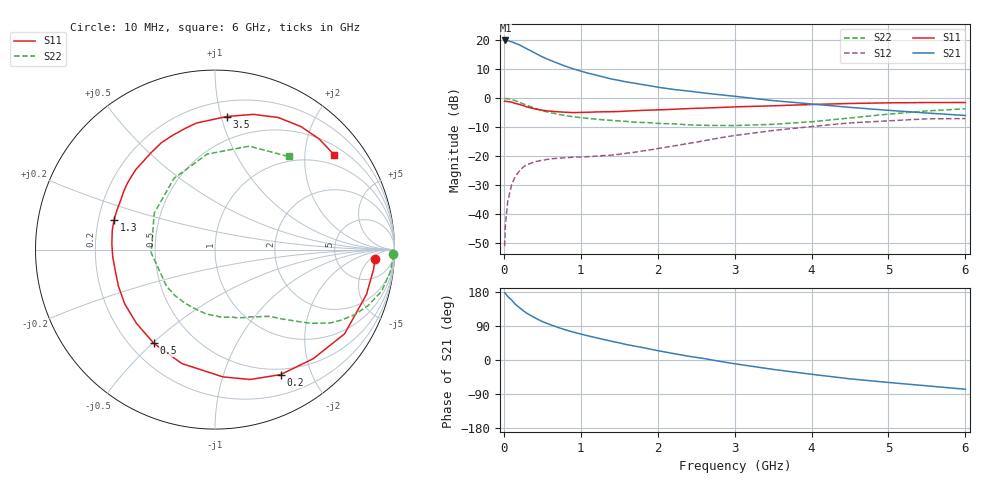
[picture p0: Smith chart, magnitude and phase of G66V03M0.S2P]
! SIEMENS Small Signal Semiconductors
! BFG193
! Si NPN RF Bipolar Junction Transistor in SOT223
! VCE = 6 V  IC = 3 mA
! Common Emitter S-Parameters:  August  1996
# GHz  S  MA  R  50
!  f  S11  S21  S12  S22
! GHz  MAG  ANG  MAG  ANG  MAG  ANG  MAG  ANG
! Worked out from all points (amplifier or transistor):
!   36 points, 10 MHz to 6 GHz, reference 50 ohm
!   highest |S21| = 20.0 dB at 20 MHz (marker M1)
!   |S21| within 3 dB of that: start of sweep to 306.8 MHz
!   unconditionally stable (mu >= 1): 1.291 GHz to 2.519 GHz
!   at 250 MHz: K = 0.23, MSG = 20.8 dB, |S12| = -23.8 dB
!   at 1.4 GHz: K = 1.07, MAG = 11.5 dB, |S12| = -19.6 dB
!   at 6 GHz: K = 0.90, MSG = 0.5 dB, |S12| = -7.0 dB
!   S11 on the Smith chart (normalised r, x): 10 MHz: 14, -7; 200 MHz: 0.43, -1.57; 500 MHz: 0.30, -0.50; 1.3 GHz: 0.27, +0.13; 3.5 GHz: 0.31, +1.04; 6 GHz: 0.71, +2.69
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0.01  0.8936 -3.3  9.914 177.4  0.0028 91.7  0.9942 -1.5
0.02  0.8907 -6.9  9.998 176.1  0.0065 84.2  0.9929 -2.9
0.05  0.8802 -16.5  9.887 167.8  0.0164 80.5  0.9847 -7.2
0.1  0.8611 -33.0  9.501 158.4  0.0317 72.7  0.9567 -14.0
0.15  0.8179 -48.0  8.935 147.0  0.0452 64.4  0.9083 -20.1
0.2  0.7866 -62.3  8.416 138.7  0.0553 58.4  0.8594 -24.9
0.25  0.7498 -74.8  7.774 130.4  0.0649 52.2  0.8054 -29.2
0.3  0.7108 -86.4  7.154 123.3  0.0712 48.0  0.7611 -32.5
0.4  0.6611 -106.3  6.113 111.8  0.0801 40.5  0.6746 -37.5
0.5  0.6234 -123.2  5.206 101.5  0.0854 35.4  0.612 -40.9
0.6  0.6002 -136.8  4.567 93.5  0.0899 32.2  0.5685 -43.6
0.7  0.587 -149.0  4.039 86.2  0.0924 30.1  0.5335 -46.3
0.8  0.5752 -159.3  3.592 79.7  0.0944 28.9  0.5038 -48.6
1.1  0.5755 176.8  2.71 63.5  0.0985 28.3  0.4495 -56.2
1.3  0.5865 163.7  2.329 54.1  0.1028 29.9  0.4249 -61.7
1.6  0.6031 147.5  1.911 40.5  0.1129 32.3  0.399 -72.2
2.2  0.647 123.3  1.428 17.2  0.15 34.7  0.3627 -97.6
2.8  0.6951 103.9  1.158 -3.3  0.2067 29.3  0.3399 -130.7
3.5  0.7441 85.0  0.914 -24.8  0.2785 15.3  0.3557 -177.1
4.5  0.816 64.4  0.699 -49.7  0.3768 -7.1  0.4577 120.0
5.5  0.8467 46.7  0.558 -68.2  0.4429 -35.2  0.6069 71.7
6  0.8483 38.6  0.506 -77.2  0.4479 -50.6  0.6611 51.7
